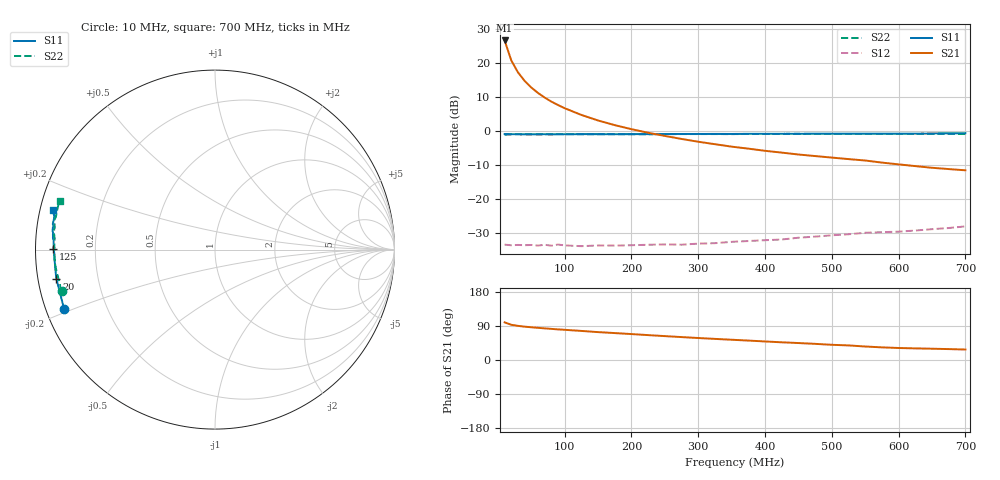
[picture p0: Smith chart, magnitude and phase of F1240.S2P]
! Date: Mon Aug 07 15:55:53 1995
# MHZ  S  MA  R  50.0000
!  POLYFET RF DEVICES
!  F1240
!  S PARAMETERS
!  VDS=28V, IDQ=600mA
!FREQ  S11MAG S11ANG S21MAG S21ANG S12MAG S12ANG S22MAG S22ANG
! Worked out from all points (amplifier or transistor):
!   34 points, 10 MHz to 700 MHz, reference 50 ohm
!   highest |S21| = 26.6 dB at 10 MHz (marker M1)
!   |S21| within 3 dB of that: start of sweep to 15.12 MHz
!   unconditionally stable (mu >= 1): 245.2 MHz to end of sweep
!   at 60 MHz: K = 0.26, MSG = 22.4 dB, |S12| = -33.6 dB
!   at 300 MHz: K = 1.16, MAG = 12.5 dB, |S12| = -33.0 dB
!   at 700 MHz: K = 1.42, MAG = 4.4 dB, |S12| = -28.0 dB
!   S11 on the Smith chart (normalised r, x): 10 MHz: 0.05, -0.19; 20 MHz: 0.05, -0.09; 125 MHz: 0.05, +0.00; 700 MHz: 0.04, +0.12
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10  0.9032 -158.6  21.26 99.4  0.02159 12.0  0.8848 -164.8
20  0.8987 -169.5  10.84 92.9  0.02116 6.8  0.8919 -172.7
30  0.8965 -173.2  7.239 90.1  0.0214 6.4  0.8953 -175.5
40  0.8954 -175.2  5.428 88.0  0.02119 5.3  0.894 -177.0
50  0.896 -176.5  4.341 86.4  0.02137 6.3  0.8949 -178.0
60  0.8961 -177.4  3.613 84.9  0.02096 6.3  0.8938 -178.9
70  0.897 -178.0  3.095 83.5  0.02149 8.0  0.8945 -179.5
80  0.8956 -178.7  2.699 82.1  0.02086 6.5  0.8947 -179.7
90  0.8969 -179.2  2.404 80.8  0.02167 6.9  0.8956 179.7
100  0.8972 -179.6  2.159 79.7  0.02106 8.0  0.8942 179.4
125  0.9005 179.7  1.721 76.7  0.02052 7.4  0.8952 178.3
150  0.8996 178.8  1.427 73.6  0.02103 9.3  0.895 177.6
175  0.8991 178.3  1.22 71.1  0.02091 13.9  0.8977 177.0
200  0.9005 177.6  1.064 68.4  0.02118 16.3  0.895 176.2
225  0.9005 176.8  0.9429 65.7  0.02151 18.6  0.8984 175.3
250  0.9028 176.4  0.8471 63.0  0.02179 21.4  0.899 174.8
300  0.9059 175.2  0.6964 58.0  0.02237 26.5  0.9025 173.3
375  0.9095 173.7  0.5518 51.3  0.02441 32.7  0.905 171.3
475  0.9149 171.1  0.4296 42.6  0.02832 39.5  0.9057 168.6
550  0.9131 169.3  0.3698 35.6  0.03226 42.6  0.9068 166.6
600  0.9137 168.3  0.3247 31.7  0.03348 43.7  0.9067 165.4
700  0.9288 166.1  0.2656 27.6  0.04002 46.5  0.9032 162.4
